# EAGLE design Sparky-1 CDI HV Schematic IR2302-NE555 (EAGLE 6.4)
Miniature low power CDi for RC and other small battery powered engines.
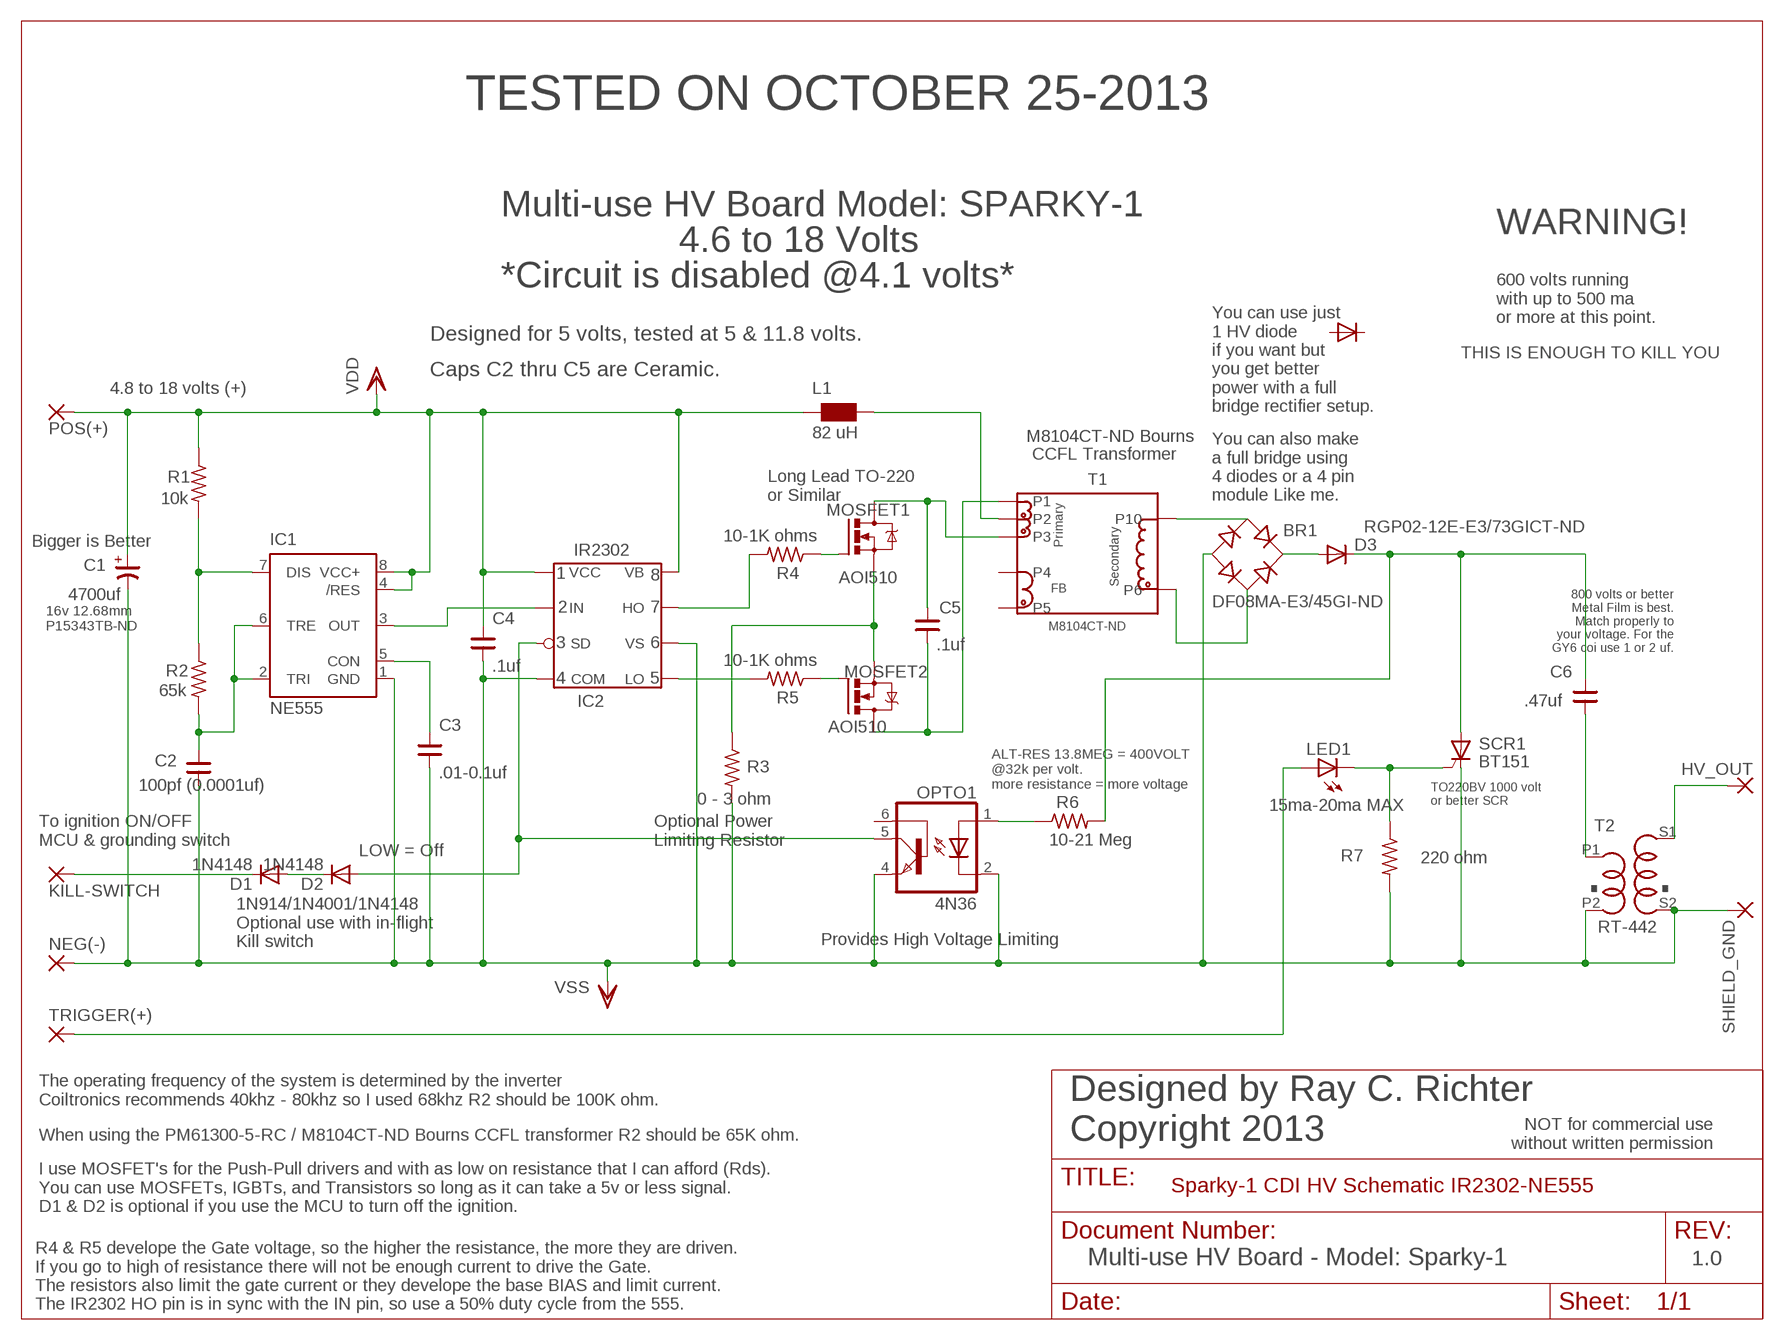
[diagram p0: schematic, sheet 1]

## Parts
BR1  DF08MA-E3/45GI-ND  B-DIL  [B-DIL]
C1  4700uf  CP-E-075X160  [E-075X160]
C2  100pf (0.0001uf)  CNP-C050-075X030  [C050-075X030]
C3  .01-0.1uf  CNP-C050-075X030  [C050-075X030]
C4  .1uf  CNP-C050-075X030  [C050-075X030]
C5  .1uf  CNP-C050-075X030  [C050-075X030]
C6  .47uf  CNP-C275-320X100  [C275-320X100]
D1  1N4148  [RAD2,5L]
D2  1N4148  [RAD2,5L]
D3  RGP02-12E-E3/73GICT-ND  DIODE-C1702-05  [C1702-05]
HV_OUT  3,81/1,1  [3,81/1,1]
IC1  NE555  [DIL-08]
IC2  IR2302  [DIL8]
KILL-SWITCH  2,54/0,8  [2,54/0,8]
L1  82 uH  WE-TI_L  [WE-TI_L]
LED1  15ma-20ma MAX  LED5MM  [LED5MM]
MOSFET1  AOI510  IRF520  [TO220BV]
MOSFET2  AOI510  IRF520  [TO220BV]
NEG(-)  2,54/0,8  [2,54/0,8]
OPTO1  4N36  4N37M  [DIL06]
POS(+)  2,54/0,8  [2,54/0,8]
R1  10k  R-US_0207/2V  [0207/2V]
R2  65k  R-US_0207/2V  [0207/2V]
R3  0 - 3 ohm  R-US_0204/7  [0204/7]
R4  10-1K ohms  R-US_0207/2V  [0207/2V]
R5  10-1K ohms  R-US_0204/7  [0204/7]
R6  10-21 Meg  R-US_0207/2V  [0207/2V]
R7  220 ohm  R-US_0204/7  [0204/7]
SCR1  BT151  BT151TO220BV  [TO220BV]
SHIELD_GND  3,81/1,1  [3,81/1,1]
T1  M8104CT-ND  CCFL-INVERTERCCFL-INVERTER-SMD  [CCFL-INVERTER_SMD]
T2  RT-442  [RT-442]
TRIGGER(+)  2,54/0,8  [2,54/0,8]

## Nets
N$2: LED1.A TRIGGER(+).1(P)
N$3: C6.2 D3.C R6.2 SCR1.A
N$4: BR1.AC2 T1.P$6(P6)
N$5: C5.2 MOSFET1.D T1.P$3(P3)
N$6: BR1.+ D3.A
N$7: MOSFET2.G R5.1
N$8: MOSFET1.G R4.1
N$9: IC2.P$5(LO) R5.2
N$10: IC2.P$7(HO) R4.2
N$11: BR1.AC1 T1.P$10(P10)
N$12: LED1.K(C) R7.1 SCR1.G
N$14: OPTO1.1(A) R6.1
N$15: IC1.3(OUT) IC2.P$2(IN)
N$16: D2.A IC2.P$3(SD) OPTO1.5(COL)
N$17: HV_OUT.1(P) T2.S1
N$18: C5.1 MOSFET2.D T1.P$1(P1)
N$19: C3.2 IC1.5(CON)
N$21: C6.1 T2.P1
N$22: C2.2 IC1.2(TRI) IC1.6(TRE) R2.2
N$23: D1.C KILL-SWITCH.1(P)
N$24: IC1.7(DIS) R1.2 R2.1
N$25: D1.A D2.C
N$26: MOSFET1.S MOSFET2.S R3.1
VDD: C1.+ C4.2 IC1.4(/RES) IC1.8(VCC+) IC2.P$1(VCC) IC2.P$8(VB) L1.1 L1.2 POS(+).1(P) R1.1 T1.P$2(P2)
VSS: BR1.- C1.- C2.1 C3.1 C4.1 IC1.1(GND) IC2.P$4(COM) IC2.P$6(VS) NEG(-).1(P) OPTO1.2(C) OPTO1.4(EMI) R3.2 R7.2 SCR1.K SHIELD_GND.1(P) T2.P2 T2.S2
Unconnected: OPTO1.6(BAS) T1.P$4(P4) T1.P$5(P5)

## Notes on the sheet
- TESTED ON OCTOBER 25-2013
- Multi-use HV Board Model: SPARKY-1
- WARNING!
- 4.6 to 18 Volts
- *Circuit is disabled @4.1 volts*
- 600 volts running
  with up to 500 ma 
  or more at this point.
- Designed for 5 volts, tested at 5 & 11.8 volts.
- THIS IS ENOUGH TO KILL YOU
- Caps C2 thru C5 are Ceramic.
- 4.8 to 18 volts (+)
- You can use just
  1 HV diode
  if you want but
  you get better
  power with a full
  bridge rectifier setup.
- M8104CT-ND Bourns
- CCFL Transformer
- Long Lead TO-220
  or Similar
- You can also make
  a full bridge using
  4 diodes or a 4 pin
  module Like me.
- Bigger is Better
- 800 volts or better
  Metal Film is best.
  Match properly to
  your voltage. For the
  GY6 coi use 1 or 2 uf.
- 16v 12.68mm
  P15343TB-ND
- ALT-RES 13.8MEG = 400VOLT
  @32k per volt. 
  more resistance = more voltage
- TO220BV 1000 volt
  or better SCR
- To ignition ON/OFF
  MCU & grounding switch
- Optional Power
  Limiting Resistor
- LOW = Off
- Provides High Voltage Limiting
- 1N914/1N4001/1N4148
  Optional use with in-flight
  Kill switch
- The operating frequency of the system is determined by the inverter 
  Coiltronics recommends 40khz - 80khz so I used 68khz R2 should be 100K ohm.
- NOT for commercial use
  without written permission
- When using the PM61300-5-RC / M8104CT-ND Bourns CCFL transformer R2 should be 65K ohm.
- Designed by Ray C. Richter
  Copyright 2013
- I use MOSFET's for the Push-Pull drivers and with as low on resistance that I can afford (Rds). 
  You can use MOSFETs, IGBTs, and Transistors so long as it can take a 5v or less signal.
  D1 & D2 is optional if you use the MCU to turn off the ignition.
- Multi-use HV Board - Model: Sparky-1 | 1.0
- R4 & R5 develope the Gate voltage, so the higher the resistance, the more they are driven. 
  If you go to high of resistance there will not be enough current to drive the Gate.
  The resistors also limit the gate current or they develope the base BIAS and limit current.
  The IR2302 HO pin is in sync with the IN pin, so use a 50% duty cycle from the 555.

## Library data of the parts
BR1 = rectifier:B-DIL: RECTIFIER
C1 = cap-master:CP-: POLARIZED CAP
C2-C6 = cap-master:CNP-: NON-POLARIZED CAP
D1 D2 = diode:1N4148: DIODE
D3 = diode:DIODE-: DIODE
HV_OUT SHIELD_GND = wirepad:3,81/1,1: THROUGH-HOLE PAD
IC1 = st-microelectronics:NE555: General purpose bipolar Timer; MF: Arrow Electronics; MPN: NE555N; OC_FARNELL: 1467742; OC_NEWARK: 89K1486
IC2 = MY-Custom:IR2302
KILL-SWITCH NEG(-) POS(+) TRIGGER(+) = wirepad:2,54/0,8: THROUGH-HOLE PAD
L1 = wuerth-elektronik:WE-TI: Radial Leaded Wire Wound Inductor WE-TI
LED1 = led:LED: LED
MOSFET1 MOSFET2 = transistor-power:IRF520: HEXFET Power MOSFET
OPTO1 = optocoupler:4N*?M: General Purpose 6-Pin Phototransistor Optocouplers Source: http://www.fairchildsemi.com/ds/4N/4N35-M.pdf; MPN: 4N37-M; OC_FARNELL: 1021353; OC_NEWARK: 98K9125
R1-R7 = R-C-L-E:R-US_: RESISTOR, American symbol
SCR1 = triac:BT151: THYRISTOR
T1 = MY_STUFF:CCFL-INVERTER; MANUFACTURER: Cooper Bussmann
T2 = MY-Custom:RT-442

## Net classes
0 default: clearance 0.355 mm

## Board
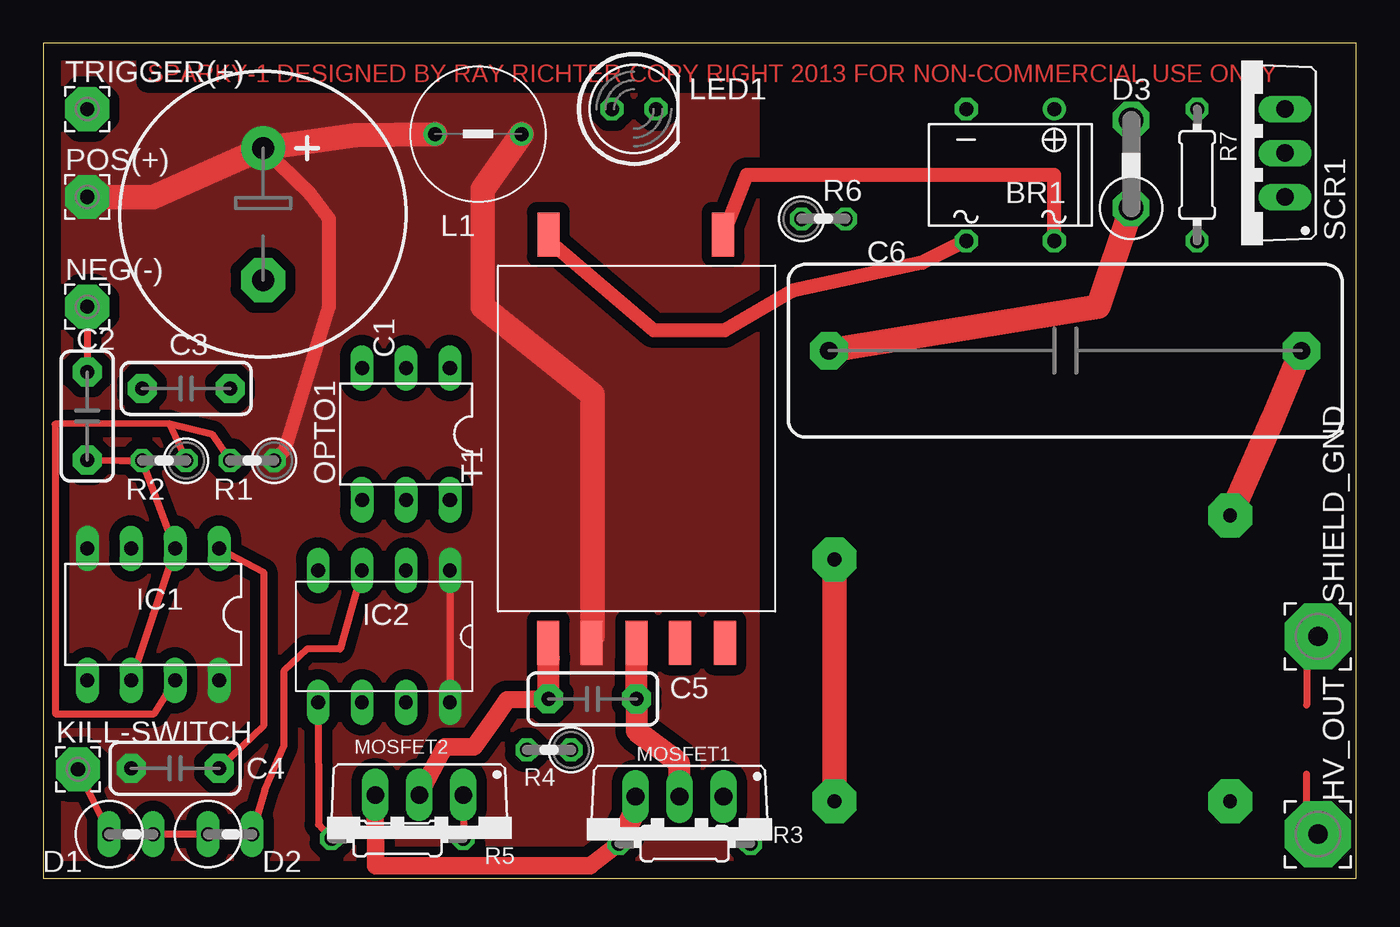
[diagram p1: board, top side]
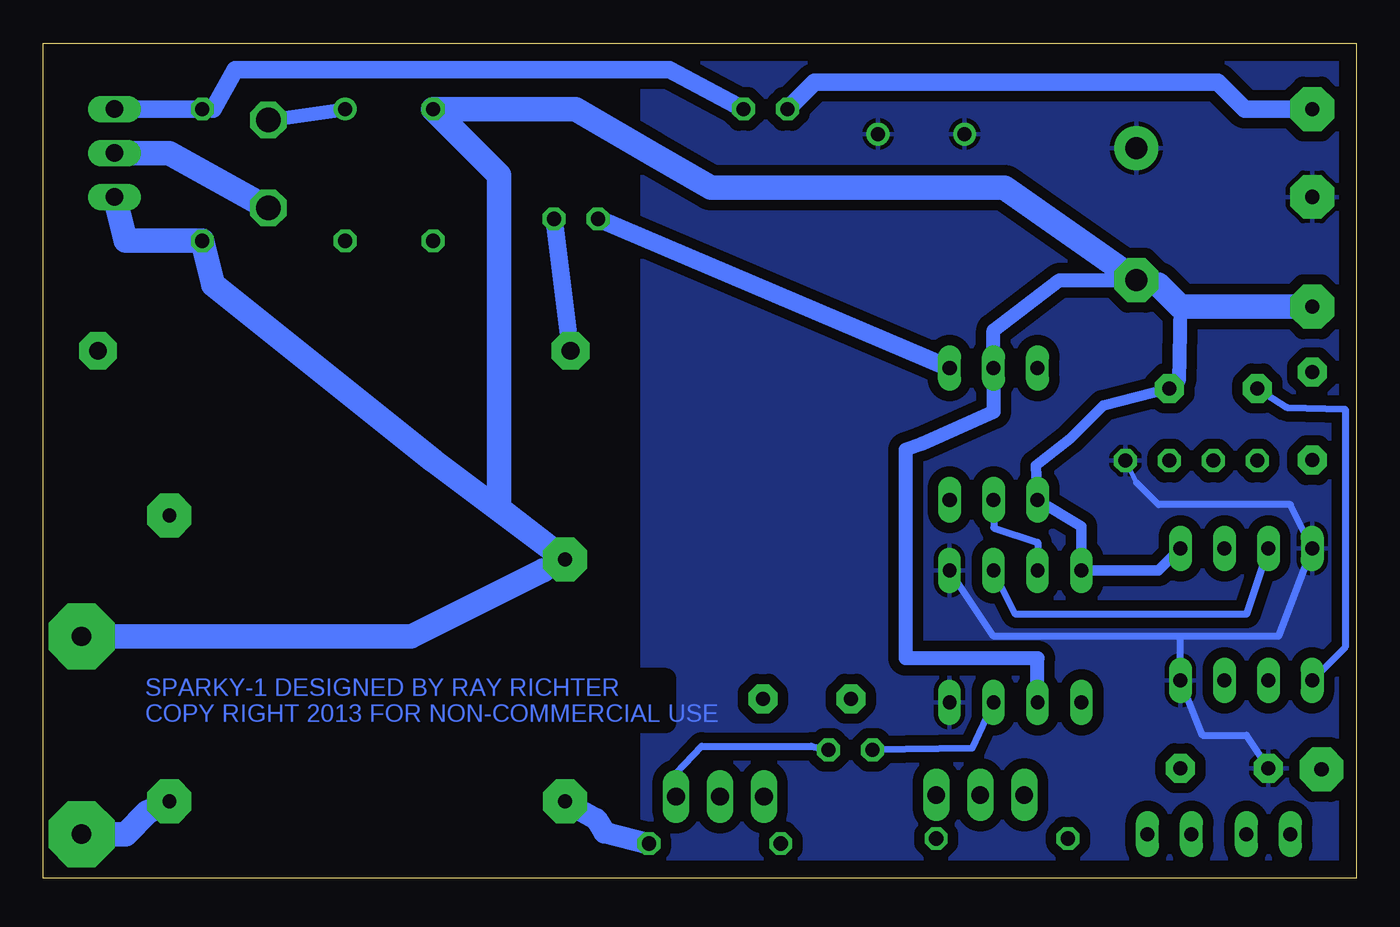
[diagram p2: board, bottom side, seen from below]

Size 75.87 x 48.25 mm. Coordinates in mm from the lower left corner, seen from the top.
Outline: 0,0 75.87,0 75.87,48.25 0,48.25 0,0
Copper layers (1*16): Top 0.035mm / dielectric 1.5mm / Bottom 0.035mm
Design rules "Sparky-1 CDI HV Schematic IR2302-NE555": minimum track width 10mil, minimum drill 24mil, track to track 0.355mm, track to pad 0.355mm, pad to pad 0.355mm, via to via 0.355mm, smd to smd 8mil, copper to edge 40mil, drill to drill 8mil, minimum pad ring 10mil, minimum via ring 8mil, stop-mask expansion 4mil, vias tented up to drill 0mil, thermal gap 10mil
tRestrict: area 42,0 to 76,48
bRestrict: area 42,0 to 76,48

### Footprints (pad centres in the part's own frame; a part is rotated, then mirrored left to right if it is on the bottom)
B-DIL = drill 0.813: + -2.54,-3.81 | drill 0.813 octagon: - 2.54,-3.81; AC1 2.54,3.81; AC2 -2.54,3.81
E-075X160 = drill 1.27 pad 2.54: + -3.81,0 | drill 1.27 pad 2.54 octagon: - 3.81,0
C050-075X030 = drill 0.813 pad 1.676 octagon: 1 -2.54,0; 2 2.54,0
C275-320X100 = drill 1.016 pad 2.184 octagon: 1 -13.652,0; 2 13.652,0
RAD2,5L = drill 0.813 long: A 1.27,0; C -1.27,0
C1702-05 = drill 1.397 octagon: A 2.54,0; C -2.54,0
3,81/1,1 = drill 1.118 pad 3.81 octagon: 1 0,0
DIL-08 = drill 0.813 long: 1 -3.81,-3.81; 2 -1.27,-3.81; 3 1.27,-3.81; 4 3.81,-3.81; 5 3.81,3.81; 6 1.27,3.81; 7 -1.27,3.81; 8 -3.81,3.81
DIL8 = drill 0.8 long: P$1 -3.81,3.81; P$2 -3.81,1.27; P$3 -3.81,-1.27; P$4 -3.81,-3.81; P$5 3.81,-3.81; P$6 3.81,-1.27; P$7 3.81,1.27; P$8 3.81,3.81
2,54/0,8 = drill 0.813 pad 2.54 octagon: 1 0,0
WE-TI_L = drill 0.813: 1 -2.5,0; 2 2.5,0
LED5MM = drill 0.813 octagon: A -1.27,0; K 1.27,0
TO220BV = drill 1.016 long: D 0,-2.54; G -2.54,-2.54; S 2.54,-2.54
DIL06 = drill 0.813 long: 1 -2.54,-3.81; 2 0,-3.81; 3 2.54,-3.81; 4 2.54,3.81; 5 0,3.81; 6 -2.54,3.81
0207/2V = drill 0.813 octagon: 1 -1.27,0; 2 1.27,0
0204/7 = drill 0.813 octagon: 1 -3.81,0; 2 3.81,0
TO220BV' = drill 1.016 long: A 0,-2.54; G 2.54,-2.54; K -2.54,-2.54
CCFL-INVERTER_SMD = smd 2.54 x 1.27: P$1 -11.8,5.11; P$2 -11.8,2.6; P$3 -11.8,0; P$4 -11.8,-2.5; P$5 -11.8,-5.1; P$6 11.8,-5; P$10 11.8,5.1
RT-442 = drill 0.8 pad 2.54 octagon: P1 11.43,8.255; P2 -11.43,5.715; S1 11.43,-8.255; S2 -11.43,-8.255

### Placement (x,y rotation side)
BR1  55.88,40.64 180 top
C1  12.7,38.37 270 top
C2  2.54,26.7 270 top
C3  8.26,28.3 180 top
C4  7.62,6.35 180 top
C5  31.75,10.36 0 top
C6  59.05,30.48 180 top
D1  5.08,2.54 0 top
D2  10.79,2.54 0 top
D3  62.87,41.27 90 top
HV_OUT  73.66,2.54 0 top
IC1  6.35,15.24 180 top
IC2  19.68,13.97 270 top
KILL-SWITCH  2,6.29 0 top
L1  25.13,43 180 top
LED1  34.13,44.45 0 top
MOSFET1  36.77,2.17 180 top
MOSFET2  21.73,2.27 180 top
NEG(-)  2.54,33.02 0 top
OPTO1  20.95,25.67 180 top
POS(+)  2.54,39.37 0 top
R1  12.06,24.13 180 top
R2  6.99,24.13 180 top
R3  37.06,2 0 top
R4  29.22,7.41 180 top
R5  20.46,2.29 180 top
R6  45.09,38.1 0 top
R7  66.67,40.64 270 top
SCR1  BT151  [TO220BV']  69.22,41.91 90 top
SHIELD_GND  73.66,13.97 0 top
T1  34.29,25.4 90 top
T2  57.15,12.7 0 top
TRIGGER(+)  2.54,44.45 0 top

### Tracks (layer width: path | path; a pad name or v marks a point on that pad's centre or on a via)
N$2
  Bottom 1.016: TRIGGER(+).1 6.45,44.45 8,46 19,46 31.31,46 LED1.A
N$3
  Top 1.422: D3.C 60.96,33.02 C6.2
  Bottom 1.016: R6.2 C6.2
  Bottom 1.422: SCR1.A 68.58,41.91 D3.C
N$4
  Top 0.813: BR1.AC2 58.42,40.64 40.64,40.64 T1.P$6
N$5
  Top 0.254: 34.29,10.16 C5.2 | 34.29,12.7 T1.P$3 | 34.29,10.16 C5.2 | 34.29,10.16 C5.2
  Top 1.27: C5.2 34.29,12.7 | 34.29,10.16 34.29,8.52 36.73,6.68 MOSFET1.D
N$6
  Bottom 0.813: D3.A BR1.+
N$7
  Top 0.406: MOSFET2.G R5.1
N$8
  Bottom 0.406: R4.1 31.48,7.62 37.83,7.62 39.27,6.08 MOSFET1.G
N$9
  Top 0.406: IC2.P$5 15.9,3.1 R5.2
N$10
  Bottom 0.406: IC2.P$7 22.2,7.5 R4.2
N$11
  Top 0.254: 29.21,36.83 T1.P$10
  Top 0.813: 29.21,36.83 35.29,31.66 39.37,31.66 43.32,33.95 50.8,35.56 BR1.AC1
N$12
  Bottom 0.254: 66.04,44.45 R7.1
  Bottom 0.406: SCR1.G 72.39,44.45
  Bottom 1.016: 72.39,44.45 69.85,44.45 R7.1 | 66.04,44.45 64.77,46.72 39.67,46.72 LED1.K
N$14
  Bottom 1.016: R6.1 OPTO1.1
N$15
  Bottom 0.406: IC2.P$2 19.68,15.24 6.35,15.24 IC1.3
N$16
  Top 0.406: D2.A 12.43,3.81 12.8,5.08 13.9,7.62 13.9,11.97 15.24,13.24 17.14,13.24 IC2.P$3
  Bottom 0.406: OPTO1.5 20.95,20.25 18.4,19.4 IC2.P$3
N$17
  Bottom 1.422: HV_OUT.1 71.12,2.54 69.85,3.81 T2.S1
N$18
  Top 0.254: 29.21,12.7 T1.P$1 | 29.21,10.16 C5.1
  Top 1.016: MOSFET2.D 23.2,7.6 24.9,7.6 26.2,9.4 26.8,10.3 C5.1
  Top 1.27: C5.1 29.21,12.7
N$19
  Bottom 0.406: C3.2 4.01,27.2 0.64,27.1 0.64,13.34 IC1.5
N$21
  Top 1.422: T2.P1 71.12,26.67 C6.1
N$22
  Top 0.406: C2.2 4.45,24.13 R2.2 IC1.2 6.35,15.24 IC1.6
N$23
  Top 0.406: KILL-SWITCH.1 D1.C
N$24
  Top 0.254: 7.29,26.26 R2.1
  Top 0.406: IC1.7 6.4,9.5 0.7,9.5 0.69,26.24 7.29,26.26 | 7.29,26.26 9.76,25.66 R1.2 | 7.29,26.26 R2.1
N$25
  Top 0.254: 5.08,2.54 D1.A
  Top 0.406: D2.C 5.08,2.54
N$26
  Top 0.254: 34.19,3.91 34.12,3.74
  Top 1.016: MOSFET2.S 19.2,0.7 31.6,0.7 R3.1
  Top 1.27: 34.12,3.74 R3.1 | 34.19,3.91 MOSFET1.S
N$27
  Top 0.406: 74,14 73,14 73,10
N$28
  Top 0.406: 74,3 73,3 73,6
VDD
  Top 0.254: 31.75,13.97 T1.P$2
  Top 0.406: IC2.P$1 IC2.P$8
  Top 0.813: C1.+ 15.44,39.52 16.51,38.1 16.51,33.02 13.97,24.77 R1.1
  Top 1.422: POS(+).1 6.35,39.37 C1.+ 18.02,42.94 L1.2 | 31.75,13.97 31.75,27.94 25.4,33.02 25.4,39.8 L1.1
  Bottom 0.254: 12.7,22.86 R1.1
  Bottom 0.406: 12.7,22.86 11.43,21.59 3.81,21.59 IC1.4 4.48,13.97 10.16,13.97 | IC2.P$1 20.95,13.97 10.16,13.97 | 10.16,13.97 IC1.8 8.89,8.26 6.35,8.26 C4.2
  pour Top (isolate 0.61, no thermals): 0,48 76,48 76,0 0,0
  pour Bottom (isolate 0.61): 0,48 76,48 76,0 0,0
VSS
  Top 0.406: NEG(-).1 C2.1 | C4.1 12.73,8.79 12.73,17.68 IC1.1
  Top 1.422: T2.P2 T2.S2
  Bottom 0.254: 45.72,4.41 T2.S2
  Bottom 0.406: 46.99,17.78 T2.P2
  Bottom 0.61: IC1.1 11.43,17.78 IC2.P$4 15.88,20.32 OPTO1.4 18.51,23.86 16.51,25.4 14.61,27.3 C3.1
  Bottom 0.813: IC2.P$6 18.41,12.7 26.04,12.7 26.04,24.77 25.1,25.1 20.95,26.94 OPTO1.2 20.95,31.66 17.14,34.56 C1.- | 10.16,33.02 10.26,28.74 C3.1
  Bottom 1.27: 45.72,4.41 43.91,3.41 43.44,2.64 R3.2
  Bottom 1.422: SHIELD_GND.1 54.61,13.97 46.99,17.78 | SCR1.K 71.12,36.83 R7.2 66.04,34.29 53.34,24.13 T2.P2 49.53,21.36 49.53,40.64 BR1.- 45.1,44.45 40.76,41.89 37.29,39.91 20.32,39.91 C1.- 11.43,34.29 10.16,33.02 NEG(-).1

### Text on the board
Top: SPARKY-1 DESIGNED BY RAY RICHTER COPY RIGHT 2013 FOR NON-COMMERCIAL USE ONLY
Bottom: SPARKY-1 DESIGNED BY RAY RICHTER / COPY RIGHT 2013 FOR NON-COMMERCIAL USE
